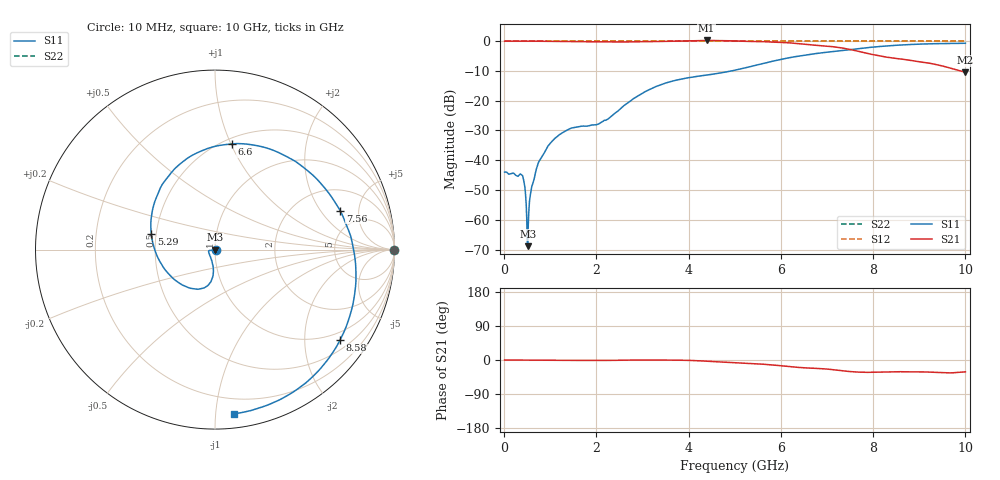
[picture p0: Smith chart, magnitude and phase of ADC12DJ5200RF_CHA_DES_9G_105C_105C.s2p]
! Texas Instruments, Inc.
! ADC12DJ5200RF - CH A S-Parameters (DES Mode, Fs = 9 GSPS, 105 degC case, 105 degC juntion)
! Port 1 represents the 100-ohm differenal input, Port 2 the digital output
! freq  dbS11  angS11  dbS21 angS21 dbS12 angS12 dbS22 angS22
# HZ S DB R 100
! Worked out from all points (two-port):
!   1000 points, 10 MHz to 10 GHz, reference 100 ohm
!   highest |S21| = 0.24 dB at 4.39 GHz (marker M1); lowest = -10.4 dB at 10 GHz (marker M2)
!   |S21| within 3 dB of the highest: start of sweep to 7.485 GHz
!   lowest |S11| = -68.9 dB at 510 MHz (marker M3), VSWR 1.00, Z = 100 - j0.0713 ohm
!   |S11| at or under -10 dB: start of sweep to 4.932 GHz
!   |S22| runs from 0.0 to 0.0 dB; largest |S21 - S12| = 0.76
!   S11 on the Smith chart (normalised r, x): 10 MHz: 1.01, -0.00; 5.29 GHz: 0.47, +0.10; 6.6 GHz: 0.55, +1.01; 7.56 GHz: 3.35, +3.13; 8.58 GHz: 0.75, -2.91; 10 GHz: 0.09, -1.12
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1e7  -43.98 -7.6  0.00 -0.0  0.00 0.0  0.00 0.0
3.8e8  -44.92 -10.5  0.01 -0.4  0.00 0.0  0.00 0.0
4.3e8  -47.24 -0.5  0.00 -0.5  0.00 0.0  0.00 0.0
4.7e8  -52.81 6.8  -0.00 -0.5  0.00 0.0  0.00 0.0
5.1e8  -68.87 -81.6  -0.00 -0.6  0.00 0.0  0.00 0.0
6e8  -48.82 -136.8  -0.00 -0.7  0.00 0.0  0.00 0.0
7.1e8  -42.37 -157.4  -0.03 -0.7  0.00 0.0  0.00 0.0
9.4e8  -35.52 -169.1  -0.03 -0.9  0.00 0.0  0.00 0.0
1.26e9  -30.80 -171.7  -0.10 -1.2  0.00 0.0  0.00 0.0
1.68e9  -28.56 -163.4  -0.19 -1.1  0.00 0.0  0.00 0.0
2.24e9  -26.25 -119.8  -0.23 -1.0  0.00 0.0  0.00 0.0
3.34e9  -14.98 -96.9  -0.09 -0.0  0.00 0.0  0.00 0.0
4.39e9  -11.39 -133.8  0.24 -3.2  0.00 0.0  0.00 0.0
5.01e9  -9.74 -174.4  0.06 -7.5  0.00 0.0  0.00 0.0
5.29e9  -8.74 165.9  -0.09 -8.9  0.00 0.0  0.00 0.0
5.9e9  -6.49 126.2  -0.34 -14.1  0.00 0.0  0.00 0.0
6.6e9  -4.49 81.1  -1.14 -21.2  0.00 0.0  0.00 0.0
6.67e9  -4.33 76.5  -1.26 -21.7  0.00 0.0  0.00 0.0
7.56e9  -2.73 17.4  -2.99 -31.1  0.00 0.0  0.00 0.0
8.34e9  -1.56 -25.8  -5.49 -31.6  0.00 0.0  0.00 0.0
8.58e9  -1.31 -35.9  -5.95 -30.9  0.00 0.0  0.00 0.0
1e10  -0.71 -83.2  -10.45 -31.3  0.00 0.0  0.00 0.0
